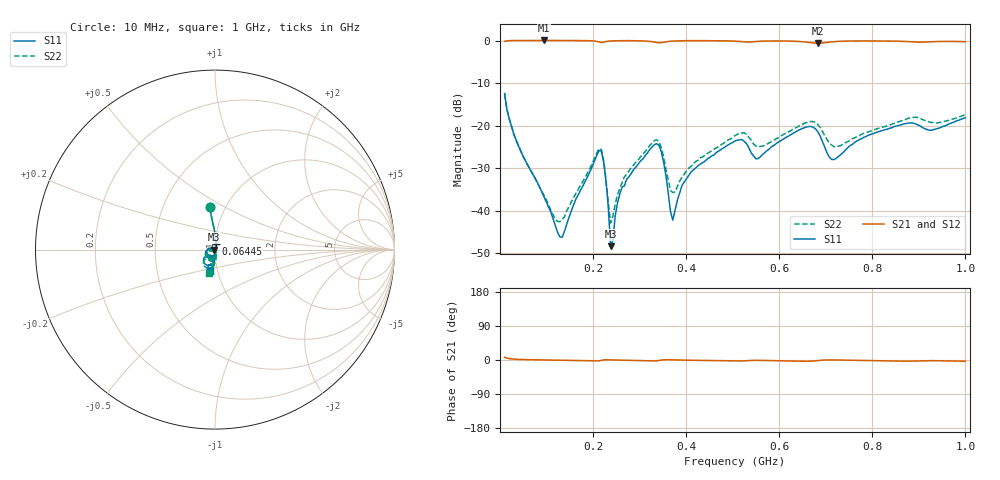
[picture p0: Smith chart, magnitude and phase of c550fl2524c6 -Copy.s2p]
!Agilent Technologies,N5234A,MY52241123,A.10.00.00
!Agilent N5234A: A.10.00.00
!Date: Monday, August 26, 2019 10:01:37
!Correction: S11(Full 2 Port(1,2))
!S21(Full 2 Port(1,2))
!S12(Full 2 Port(1,2))
!S22(Full 2 Port(1,2))
!S2P File: Measurements: S11, S21, S12, S22:
# Hz S  dB  R 50
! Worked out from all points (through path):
!   201 points, 10 MHz to 1 GHz, reference 50 ohm
!   highest |S21| = 0.02 dB at 94.15 MHz (marker M1); lowest = -0.6 dB at 683.2 MHz (marker M2)
!   lowest |S11| = -48.3 dB at 237.7 MHz (marker M3), VSWR 1.01, Z = 49.6 + j0.0535 ohm
!   |S11| at or under -10 dB: start of sweep to end of sweep
!   |S22| runs from -42.9 to -12.5 dB; largest |S21 - S12| = 0.0037
!   S11 on the Smith chart (normalised r, x): 10 MHz: 0.85, +0.42; 64.45 MHz: 1.00, +0.06; 1 GHz: 0.92, -0.22
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1e7  -12.47 97.2  -0.19 7.1  -0.19 7.2  -12.46 97.3
2.98e7  -22.04 90.4  0.00 2.3  -0.00 2.3  -21.93 90.5
6.445e7  -30.26 83.8  0.02 0.8  0.02 0.8  -30.10 82.1
9.415e7  -36.63 74.1  0.02 0.2  0.02 0.2  -36.22 67.3
1.189e8  -43.41 44.1  0.02 -0.2  0.01 -0.2  -42.08 27.6
1.3375e8  -46.21 -15.7  0.02 -0.4  0.01 -0.4  -42.06 -16.8
1.783e8  -34.11 -85.7  -0.00 -1.2  -0.01 -1.2  -33.06 -70.7
2.179e8  -26.02 -164.3  -0.47 -1.1  -0.47 -1.1  -25.59 -146.8
2.278e8  -33.02 153.2  -0.25 0.6  -0.25 0.6  -32.63 176.8
2.377e8  -48.31 171.9  -0.10 0.2  -0.10 0.2  -42.89 -143.8
2.6245e8  -34.44 -83.0  -0.03 -0.7  -0.03 -0.7  -33.40 -81.8
3.4165e8  -24.61 -157.3  -0.53 -1.2  -0.53 -1.2  -23.83 -140.7
3.7135e8  -42.21 -137.8  -0.13 0.4  -0.13 0.4  -35.73 -123.8
3.9115e8  -34.02 -85.8  -0.05 -0.3  -0.05 -0.2  -32.13 -88.2
4.1095e8  -30.84 -84.2  -0.02 -0.7  -0.03 -0.7  -29.55 -82.3
5.05e8  -23.59 -103.4  -0.14 -2.5  -0.15 -2.5  -22.34 -92.5
5.545e8  -27.74 -108.5  -0.19 -0.9  -0.20 -0.9  -24.85 -108.0
6.733e8  -20.40 -128.9  -0.56 -2.7  -0.57 -2.7  -19.06 -120.1
6.832e8  -21.46 -139.2  -0.63 -1.6  -0.63 -1.6  -19.76 -129.3
7.1785e8  -27.96 -118.0  -0.26 0.1  -0.27 0.1  -24.96 -120.1
8.3665e8  -20.64 -97.1  -0.11 -2.5  -0.13 -2.5  -19.87 -96.0
1e9  -18.14 -104.1  -0.28 -3.3  -0.28 -3.3  -17.39 -105.5
